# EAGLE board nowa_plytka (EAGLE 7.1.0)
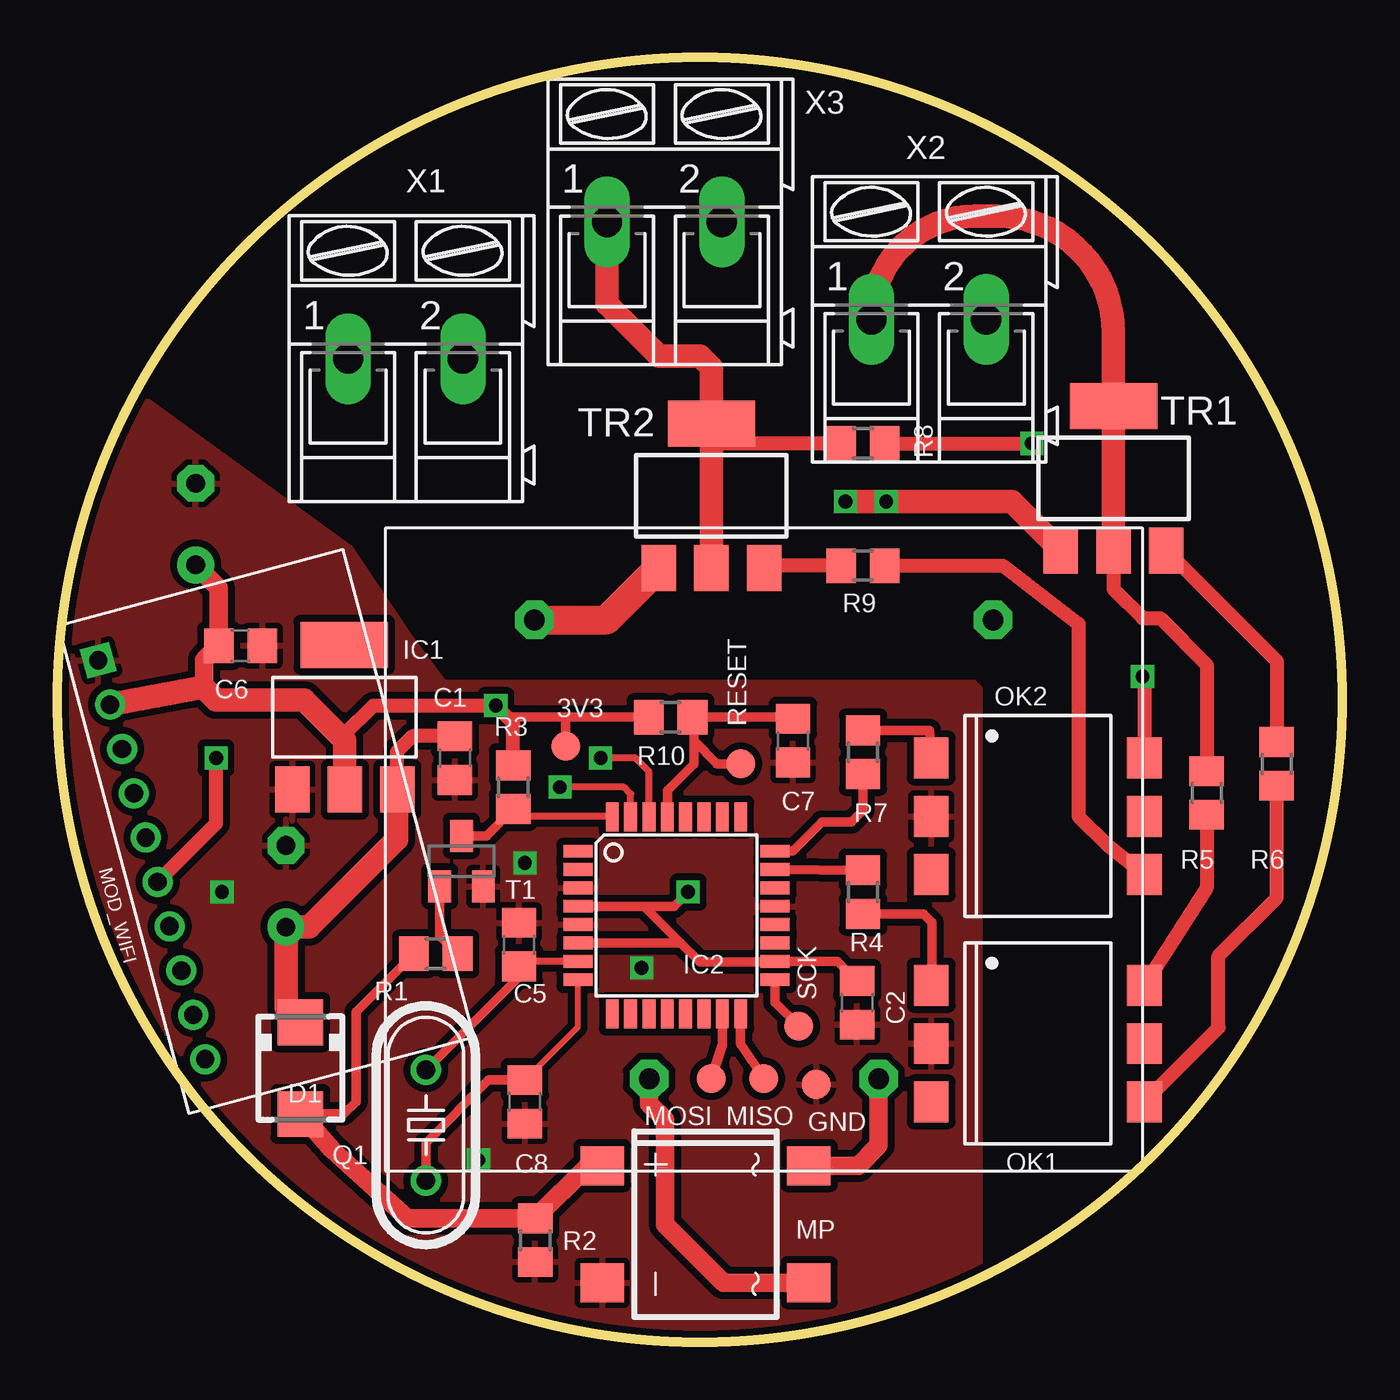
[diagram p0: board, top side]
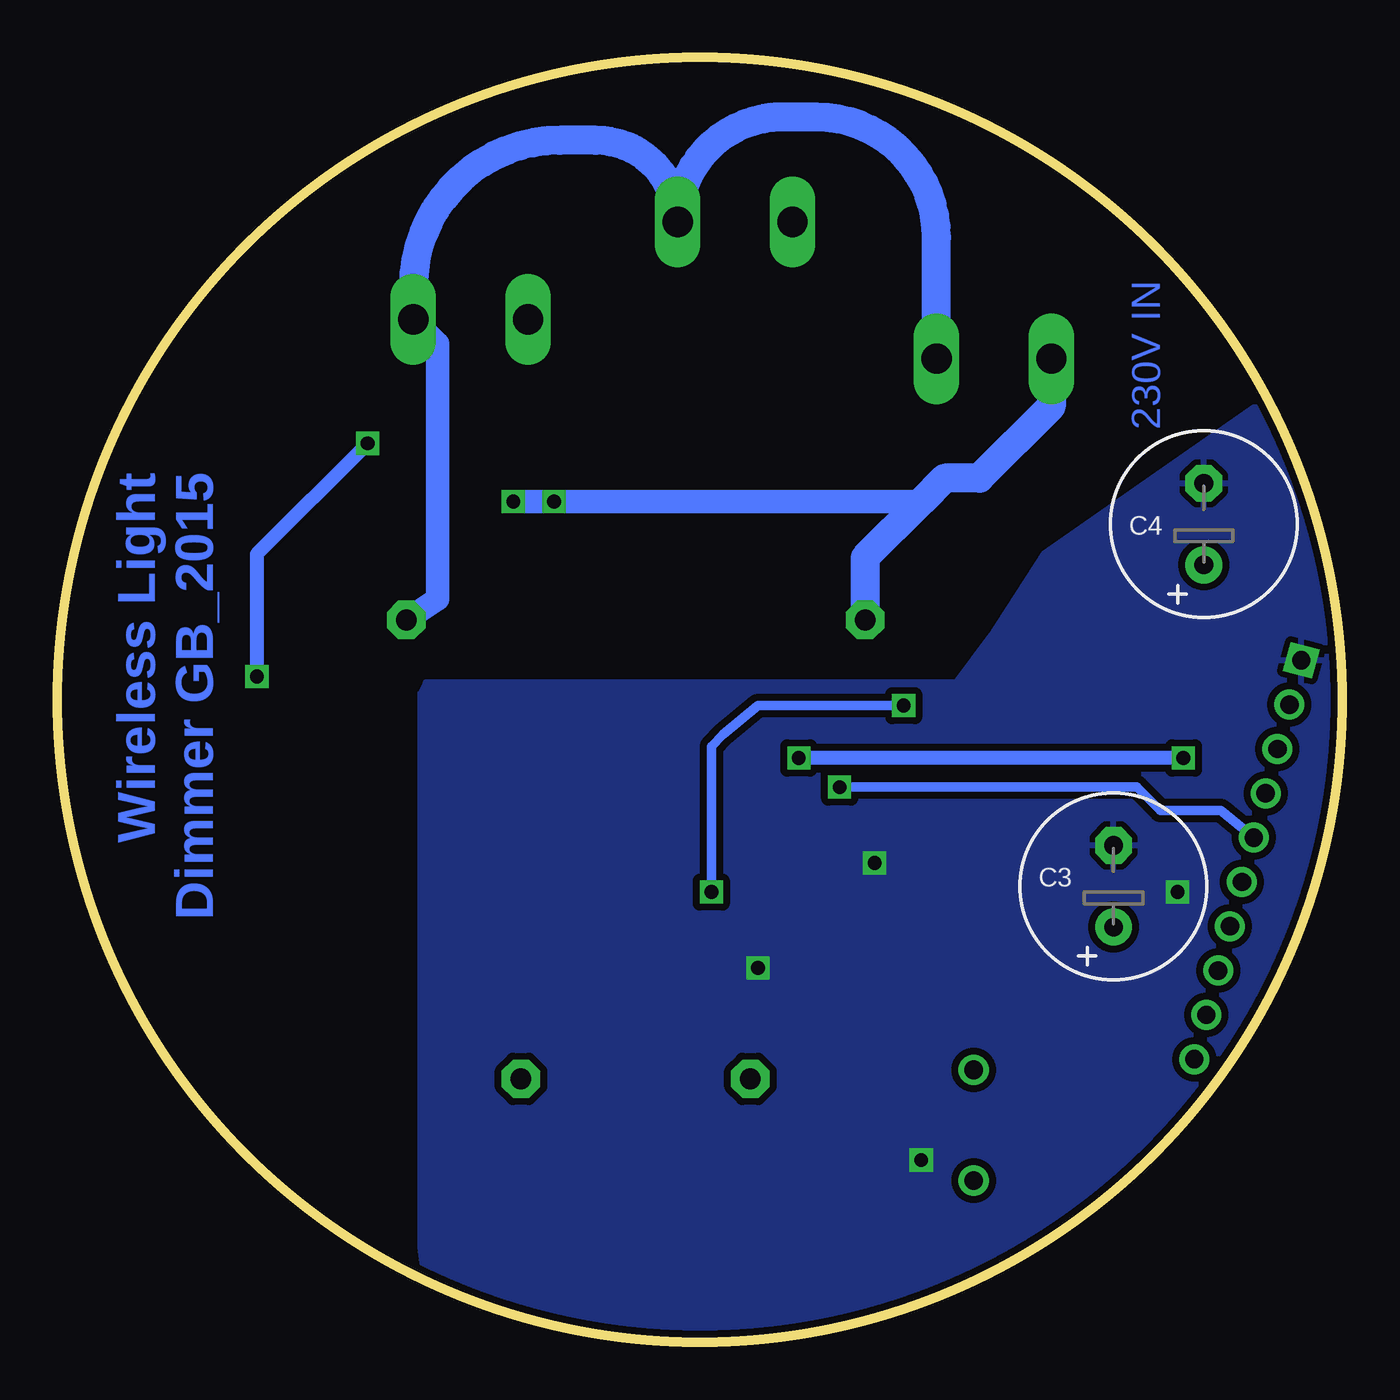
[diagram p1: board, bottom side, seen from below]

Size 56 x 56 mm. Coordinates in mm from the lower left corner, seen from the top.
Outline: circle at 28,28 radius 28
Copper layers (1*16): Top 0.035mm / dielectric 1.5mm / Bottom 0.035mm
Design rules "default *": minimum track width 10mil, minimum drill 24mil, track to track 8mil, track to pad 8mil, pad to pad 8mil, via to via 8mil, smd to smd 8mil, copper to edge 10mil, drill to drill 8mil, minimum pad ring 10mil, minimum via ring 8mil, stop-mask expansion 4mil, vias tented up to drill 0mil, thermal gap 10mil

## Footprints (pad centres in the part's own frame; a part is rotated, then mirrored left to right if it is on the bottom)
B1,27 = smd 1.27 x 1.27: TP 0,0
C0805 = smd 1.3 x 1.5: 1 -0.95,0; 2 0.95,0
E3,5-8 = drill 0.813 pad 1.6: + -1.778,0 | drill 0.813 pad 1.6 octagon: - 1.778,0
SMA = smd 2 x 2: A 2,0; C -2,0
SOT223 = smd 1.499 x 2.007: 1 -2.261,-3.15; 2 0.025,-3.15; 3 2.311,-3.15 | smd 3.81 x 2.007: 4 0,3.15
TQFP32-08 = smd 1.27 x 0.559: 1 -4.293,2.8; 2 -4.293,2; 3 -4.293,1.2; 4 -4.293,0.4; 5 -4.293,-0.4; 6 -4.293,-1.2; 7 -4.293,-2; 8 -4.293,-2.8; 17 4.293,-2.8; 18 4.293,-2; 19 4.293,-1.2; 20 4.293,-0.4; 21 4.293,0.4; 22 4.293,1.2; 23 4.293,2; 24 4.293,2.8 | smd 0.559 x 1.27: 9 -2.8,-4.293; 10 -2,-4.293; 11 -1.2,-4.293; 12 -0.4,-4.293; 13 0.4,-4.293; 14 1.2,-4.293; 15 2,-4.293; 16 2.8,-4.293; 25 2.8,4.293; 26 2,4.293; 27 1.2,4.293; 28 0.4,4.293; 29 -0.4,4.293; 30 -1.2,4.293; 31 -2,4.293; 32 -2.8,4.293
ATNEL-WIFI232-T_2 = drill 0.8 pad 1.27 square: 1 -9.1,-5.45 | drill 0.8 pad 1.27: 2 -7.1,-5.45; 3 -5.1,-5.45; 4 -3.1,-5.45; 5 -1.1,-5.45; 6 0.9,-5.45; 7 2.9,-5.45; 8 4.9,-5.45; 9 6.9,-5.45; 10 8.9,-5.45
DBS = smd 1.7 x 1.9: + -2.55,-4.5; - 2.55,-4.5; AC1 -2.55,4.5; AC2 2.55,4.5
DIL6-SMD = smd 1.78 x 1.52: 1 -2.54,-4.645; 2 0,-4.645; 3 2.54,-4.645; 4 2.54,4.645; 5 0,4.645; 6 -2.54,4.645
HC49/S = drill 0.813: 1 -2.413,0; 2 2.413,0
R0805 = smd 1.3 x 1.5: 1 -0.95,0; 2 0.95,0
SOT23 = smd 1 x 1.4: 1 -0.95,-1.1; 2 0.95,-1.1; 3 0,1.1
SOT223' = smd 1.5 x 2: 1 -2.3,-3.15; 2 0,-3.15; 3 2.3,-3.15 | smd 3.8 x 2: 4 0,3.15
TEZ1.5 = drill 0.9 pad 1.676 octagon: 1 -10,5; 2 10,5; 3 -5,-15; 4 5,-15
AK300/2 = drill 1.321 long: 1 -2.515,0; 2 2.489,0

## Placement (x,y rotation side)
3V3  TPSB1,27  [B1,27]  22.16,25.97 0 top
C1  100nF  [C0805]  17.33,25.46 90 top
C2  100nF  [C0805]  34.86,14.79 90 top
C3  470uF/10V  [E3,5-8]  9.97,19.87 90 bottom
C4  220uF/6,3V  [E3,5-8]  6.03,35.65 90 bottom
C5  22pF  [C0805]  20.13,17.33 270 top
C6  100nF  [C0805]  7.99,30.35 180 top
C7  10nF  [C0805]  32.06,26.22 270 top
C8  22pF  [C0805]  20.38,10.47 90 top
D1  S1M  [SMA]  10.59,11.94 270 top
GND  TPSB1,27  [B1,27]  33.08,11.24 0 top
IC1  REG1117  [SOT223]  12.51,27.24 0 top
IC2  MEGA8-AI  [TQFP32-08]  26.98,18.6 0 top
MISO  TPSB1,27  [B1,27]  30.79,11.49 0 top
MOD_WIFI  ATNEL-WIFI232-T_2  [ATNEL-WIFI232-T_2]  9.4,22.34 285 top
MOSI  TPSB1,27  [B1,27]  28.51,11.49 0 top
MP  [DBS]  28.25,5.14 270 top
OK1  MOC3041S  [DIL6-SMD]  42.73,13.01 270 top
OK2  MOC3041S  [DIL6-SMD]  42.73,22.92 270 top
Q1  11.0592MHz  [HC49/S]  16.06,9.46 90 top
R1  1k  [R0805]  16.49,16.93 0 top
R2  10k  [R0805]  20.83,4.44 90 top
R3  4k7  [R0805]  19.87,24.19 90 top
R4  220  [R0805]  35.11,19.62 90 top
R5  560  [R0805]  50.1,23.94 270 top
R6  560  [R0805]  53.15,25.21 270 top
R7  220  [R0805]  35.11,25.71 270 top
R8  560  [R0805]  35.11,39.18 0 top
R9  560  [R0805]  35.11,33.84 0 top
R10  10k  [R0805]  26.73,27.24 180 top
RESET  TPSB1,27  [B1,27]  29.78,25.21 0 top
SCK  TPSB1,27  [B1,27]  32.32,13.78 0 top
T1  BC847  [SOT23]  17.62,20.97 0 top
TR1  Z0103MN  [SOT223']  46.03,37.65 0 top
TR2  Z0103MN  [SOT223']  28.51,36.89 0 top
U$1  TEZ1.5/D/6V  [TEZ1.5]  30.79,26.48 0 top
X1  [AK300/2]  15.19,42.87 0 top
X2  [AK300/2]  38,44.57 0 top
X3  [AK300/2]  26.48,48.83 0 top

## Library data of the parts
3V3 GND MISO MOSI RESET SCK = testpad
C1-C8 R1-R10 = rcl
D1 = diode
IC1 = burr-brown; MPN: REG1117; OC_FARNELL: 1097566; OC_NEWARK: 14P6981
IC2 = atmel; MPN: ATMEGA8-16AU; OC_FARNELL: 9171371; OC_NEWARK: 73M8863
MOD_WIFI = ATNEL-WIFI232-T
MP = rectifier
OK1 OK2 = optocoupler; MF: FAIRCHILD SEMICONDUCTOR; MPN: MOC3041S-M; OC_FARNELL: unknown; OC_NEWARK: 05C2885
Q1 = crystal; OC_FARNELL: 1667008; OC_NEWARK: unknown
T1 = transistor
TR1 TR2 = Triac_smd
U$1 = Trafo PCB
X1-X3 = con-ptr500; OC_FARNELL: unknown; OC_NEWARK: unknown

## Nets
+3V3: 3V3.TP C2.2 C4.+ C6.2 IC1.2 IC2.4 IC2.6 IC2.18 MOD_WIFI.2 R3.2 R10.2
FAZA: TR1.1 TR2.1 U$1.1 X1.1
GND: C1.1 C2.1 C3.- C4.- C5.1 C6.1 C7.2 C8.1 GND.TP IC1.1 IC2.3 IC2.5 IC2.21 MOD_WIFI.1 MP.- OK1.2 OK2.2 R2.1 T1.2
MISO: IC2.16 MISO.TP
MOSI: IC2.15 MOSI.TP
N$1: R5.1 TR1.2 X2.1
N$2: OK2.1 R7.1
N$3: MP.AC2 U$1.3
N$4: MP.AC1 U$1.4
N$5: C1.2 C3.+ D1.C IC1.3
N$6: D1.A MP.+ R1.1 R2.2
N$7: OK1.1 R4.1
N$8: R1.2 T1.1
N$9: OK1.6 R5.2
N$10: C5.2 IC2.7 Q1.2
N$11: OK1.4 R6.2
N$12: R6.1 TR1.3
N$13: OK2.6 R8.2
N$14: OK2.4 R9.2
N$15: R9.1 TR2.3
N$16: R8.1 TR2.2 X3.1
N$17: C8.2 IC2.8 Q1.1
NEUTRAL: U$1.2 X1.2 X2.2 X3.2
OUT1: IC2.23 R4.2
OUT2: IC2.24 R7.2
RESET: C7.1 IC2.29 R10.1 RESET.TP
RXD: IC2.30 MOD_WIFI.6
SCK: IC2.17 SCK.TP
TXD: IC2.31 MOD_WIFI.5
ZERO: IC2.32 R3.1 T1.3

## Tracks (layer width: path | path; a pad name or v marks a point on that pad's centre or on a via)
+3V3  (via drill 0.6)
  Top 0.406: C2.2 34,16.6 IC2.18 31.24,16.57 28,16.57 27.17,17.4 | IC2.6 27.17,17.4 | 27.17,17.4 25.57,19 IC2.4 26.88,19 v27.49,19.62 | R10.2 22.16,27.24 | 22.16,27.24 19.62,27.24 v19.11,27.75 | 3V3.TP 22.16,27.24
  Top 0.61: 12.53,26.5 13.78,27.75 v19.11,27.75 19.87,26.98 R3.2
  Top 0.813: 12.53,26.22 12.53,26.5 | 6.41,28.51 6.41,29.72 C6.2 7.04,32.87 C4.+
  Top 1.016: IC1.2 12.53,26.22 10.75,28 6.92,28 6.41,28.51 6.37,28.55 MOD_WIFI.2
  Bottom 0.406: v27.49,19.62 27.49,25.97 26.98,26.48 25.46,27.75 v19.11,27.75
FAZA  (via drill 0.6)
  Top 1.016: TR1.1 41.6,36.64 v36.13,36.64 v34.35,36.64
  Top 1.27: U$1.1 23.94,31.48 TR2.1
  Bottom 1.016: v36.13,36.64 v34.35,36.64 18.35,36.64
  Bottom 1.27: X1.1 12.67,40.79 15.81,37.65 17.33,37.65 18.35,36.64 20.79,34.19 U$1.1
GND  (via drill 0.6)
  other vias: 7.17,19.62 25.46,16.32 18.35,7.93 20.38,20.89
  pour Top (isolate 0.305): 2.6,41.97 12.76,34.6 15.3,30.79 16.82,28.76 39.94,28.76 40.19,28.51 40.19,0.06 28.76,0.06 arc-90 -0.96,30.03
  pour Bottom (isolate 0.305): 2.09,41.97 13.01,34.35 15.3,30.79 16.82,28.76 39.94,28.76 40.19,28.25 40.19,4.12 39.68,0.31 -1.46,0.06 -1.46,38.92
MISO
  Top 0.406: IC2.16 29.78,13.01 MISO.TP
MOSI
  Top 0.406: IC2.15 28.98,12.98 MOSI.TP
N$1
  Top 0.61: TR1.2 46.03,32.83 47.3,31.56 48.07,31.56 50.1,29.52 R5.1
  Top 1.016: X2.1 arc-90 39.99,49.08 40.95,49.08 arc-90 46.03,44 TR1.2
N$2
  Top 0.406: R7.1 38.02,26.66 OK2.1
N$3
  Top 0.813: MP.AC2 29.03,2.59 26.48,5.14 26.48,9.71 25.79,10.39 U$1.3
N$4
  Top 0.813: MP.AC1 34.92,7.69 35.8,8.57 U$1.4
N$5
  Top 0.61: C1.2 15.49,26.41 14.79,25.71 14.79,24.11 IC1.3
  Top 1.016: D1.C 9.97,14.57 C3.+ 10.98,18.09 14.79,21.9 14.79,24.06 IC1.3
N$6
  Top 0.406: R1.1 13.01,14.4 13.01,10.47 12.48,9.94 D1.A
  Top 0.813: D1.A 11.97,8.39 15.26,5.39 R2.2 23.13,7.69 MP.+
N$7
  Top 0.406: R4.1 37.74,18.67 38.11,18.3 38.11,17.1 OK1.1
N$8
  Top 0.406: R1.2 16.67,17.7 T1.1
N$9
  Top 0.61: R5.2 50.1,19.8 OK1.6
N$10
  Top 0.305: IC2.7 20.35,16.6 C5.2
  Top 0.406: C5.2 20.19,16 Q1.2
N$11
  Top 0.61: OK1.4 50.61,13.7 50.61,16.82 53.15,19.36 R6.2
N$12
  Top 0.61: TR1.3 53.15,29.69 R6.1
N$13  (via drill 0.6)
  Top 0.61: R8.2 v42.48,39.18 | v47.3,29.02 47.38,28.94 OK2.6
  Bottom 0.61: v42.48,39.18 47.3,34.35 v47.3,29.02
N$14
  Top 0.61: R9.2 41.21,33.84 44.51,31.3 44.51,22.92 45.78,21.65 OK2.4
N$15
  Top 0.61: R9.1 30.91,33.84 TR2.3
N$16
  Top 0.61: R8.1 28.76,39.18 28.51,39.43
  Top 1.016: X3.1 23.96,45.25 26.22,42.99 28,42.99 28.51,42.48 28.51,39.43 TR2.2
N$17
  Top 0.254: C8.2 22.69,13.73 IC2.8
  Top 0.406: C8.2 18.79,11.42 16.06,8.7 Q1.1
NEUTRAL
  Bottom 1.016: X2.2 39.43,43.51 39.43,32.4 U$1.2
  Bottom 1.27: X1.2 17.68,48.16 arc-90 22.92,53.4 24.39,53.4 arc-90 X3.2 arc-90 32.52,52.38 34.1,52.38 arc-90 40.49,45.99 X2.2
OUT1
  Top 0.406: IC2.23 R4.2
OUT2
  Top 0.406: IC2.24 32.07,21.4 33.33,22.67 34.6,22.67 35.11,23.17 R7.2
RESET
  Top 0.406: IC2.29 26.58,24.04 27.75,25.21 27.75,26.22 | 27.75,26.22 27.75,27.17 R10.1 32,27.24 C7.1 | RESET.TP 28.76,25.21 27.75,26.22
RXD  (via drill 0.6)
  Top 0.305: IC2.30 25.78,24.88 25.21,25.46 v23.68,25.46
  Top 0.61: MOD_WIFI.6 6.92,22.61 v6.92,25.46
  Bottom 0.61: v6.92,25.46 v23.68,25.46
SCK
  Top 0.406: IC2.17 31.28,14.82 SCK.TP
TXD  (via drill 0.6)
  Top 0.305: IC2.31 24.98,23.9 24.7,24.19 v21.9,24.19
  Bottom 0.406: v21.9,24.19 8.95,24.19 7.93,23.17 5.29,23.17 MOD_WIFI.5
ZERO
  Top 0.305: 24.16,22.92 20.19,22.92 R3.1
  Top 0.406: 20.45,22.99 R3.1 18.7,22.07 T1.3 | 24.16,22.92 IC2.32

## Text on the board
Bottom: 230V IN | Wireless Light / Dimmer GB_2015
